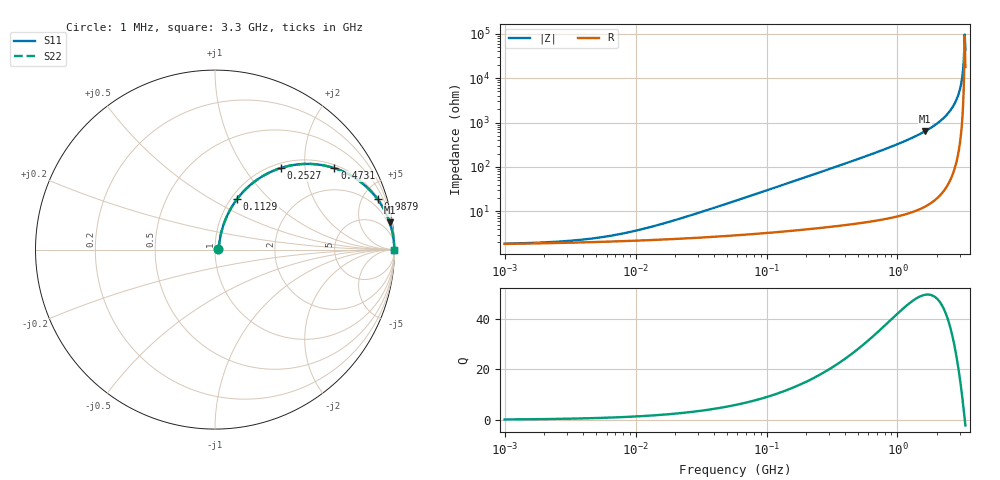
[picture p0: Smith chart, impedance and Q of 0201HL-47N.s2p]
# MHz  S  MA  R  50
!Freq  MagS11  AngS11  MagS21  AngS21  MagS12  AngS12  MagS22  AngS22
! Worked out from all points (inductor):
!   816 points, 1 MHz to 3.3 GHz, reference 50 ohm
!   read as one part in series: L = 47 nH near 25.38 MHz
!   highest Q = 49.7 at 1.625 GHz (marker M1), where L = 62.4 nH
!   self-resonance near 3.26 GHz
!   S11 on the Smith chart (normalised r, x): 1 MHz: 1.04, +0.01; 112.9 MHz: 1.07, +0.67; 252.7 MHz: 1.08, +1.50; 473.1 MHz: 1.11, +2.85; 987.9 MHz: 1.15, +6.42; 3.3 GHz: open
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1  0.01846 8.9  0.9818 -0.2  0.9818 -0.2  0.01846 8.9
3.869963  0.02265 29.0  0.9803 -0.6  0.9803 -0.6  0.02265 29.0
7.537701  0.03016 45.0  0.9789 -1.2  0.9789 -1.2  0.03016 45.0
14.97662  0.04871 60.0  0.9766 -2.5  0.9766 -2.5  0.04871 60.0
57.95895  0.1665 71.0  0.9587 -9.4  0.9587 -9.4  0.1665 71.0
112.8892  0.3088 66.3  0.9206 -17.9  0.9206 -17.9  0.3088 66.3
222.0782  0.536 54.1  0.812 -32.3  0.812 -32.3  0.536 54.1
252.7457  0.5855 51.0  0.7785 -35.8  0.7785 -35.8  0.5855 51.0
347.5104  0.7048 42.7  0.6783 -44.8  0.6783 -44.8  0.7048 42.7
473.0754  0.8053 34.3  0.564 -53.6  0.564 -53.6  0.8053 34.3
859.4345  0.9312 20.0  0.3414 -68.6  0.3414 -68.6  0.9312 20.0
987.8978  0.9484 17.2  0.2953 -71.5  0.2953 -71.5  0.9484 17.2
1624.728  0.9849 8.9  0.1545 -80.0  0.1545 -80.0  0.9849 8.9
2256.244  0.9952 4.5  0.07811 -84.2  0.07811 -84.2  0.9952 4.5
2517.22  0.997 3.1  0.05449 -85.3  0.05449 -85.3  0.997 3.1
2753.046  0.9981 2.0  0.03559 -85.9  0.03559 -85.9  0.9981 2.0
2922.414  0.9986 1.3  0.02313 -85.8  0.02313 -85.8  0.9986 1.3
3041.076  0.9988 0.8  0.01487 -85.0  0.01487 -85.0  0.9988 0.8
3102.202  0.9989 0.6  0.01075 -83.8  0.01075 -83.8  0.9989 0.6
3164.556  0.999 0.4  0.006655 -80.9  0.006655 -80.9  0.999 0.4
3293.05  0.999 -0.1  0.001916 60.2  0.001916 60.2  0.999 -0.1
3300  0.9991 -0.1  0.002305 65.6  0.002305 65.6  0.9991 -0.1
